(* Logix 5000 AddOnInstructionDefinition export Banner_IC70_PDIO_v4; software revision 33.03 *)

TYPE Banner_IC70_16P_PD_v4 :   // UDT that records the converted prcoess data.
STRUCT
   DTI : SINT[2];   // Data Transfer In
   DTO : SINT[2];   // Data Transfer Out
   PDI : Banner_IC70_16P_PDI_v4;   // Process Data In
   PDO : Banner_IC70_16P_PDO_v4;   // Process Data Out
END_STRUCT
END_TYPE

TYPE Banner_IC70_16P_PDI_v4 :
STRUCT
   C1_In : BOOL;   // Channel's current state: 0=Inactive, 1=Active
   C2_In : BOOL;   // Channel's current state: 0=Inactive, 1=Active
   C3_In : BOOL;   // Channel's current state: 0=Inactive, 1=Active
   C4_In : BOOL;   // Channel's current state: 0=Inactive, 1=Active
   C5_In : BOOL;   // Channel's current state: 0=Inactive, 1=Active
   C6_In : BOOL;   // Channel's current state: 0=Inactive, 1=Active
   C7_In : BOOL;   // Channel's current state: 0=Inactive, 1=Active
   C8_In : BOOL;   // Channel's current state: 0=Inactive, 1=Active
   C9_In : BOOL;   // Channel's current state: 0=Inactive, 1=Active
   C10_In : BOOL;   // Channel's current state: 0=Inactive, 1=Active
   C11_In : BOOL;   // Channel's current state: 0=Inactive, 1=Active
   C12_In : BOOL;   // Channel's current state: 0=Inactive, 1=Active
   C13_In : BOOL;   // Channel's current state: 0=Inactive, 1=Active
   C14_In : BOOL;   // Channel's current state: 0=Inactive, 1=Active
   C15_In : BOOL;   // Channel's current state: 0=Inactive, 1=Active
   C16_In : BOOL;   // Channel's current state: 0=Inactive, 1=Active
END_STRUCT
END_TYPE

TYPE Banner_IC70_16P_PDO_v4 :
STRUCT
   C1_Out : BOOL;   // Channel's current state: 0=Off, 1=On
   C2_Out : BOOL;   // Channel's current state: 0=Off, 1=On
   C3_Out : BOOL;   // Channel's current state: 0=Off, 1=On
   C4_Out : BOOL;   // Channel's current state: 0=Off, 1=On
   C5_Out : BOOL;   // Channel's current state: 0=Off, 1=On
   C6_Out : BOOL;   // Channel's current state: 0=Off, 1=On
   C7_Out : BOOL;   // Channel's current state: 0=Off, 1=On
   C8_Out : BOOL;   // Channel's current state: 0=Off, 1=On
   C9_Out : BOOL;   // Channel's current state: 0=Off, 1=On
   C10_Out : BOOL;   // Channel's current state: 0=Off, 1=On
   C11_Out : BOOL;   // Channel's current state: 0=Off, 1=On
   C12_Out : BOOL;   // Channel's current state: 0=Off, 1=On
   C13_Out : BOOL;   // Channel's current state: 0=Off, 1=On
   C14_Out : BOOL;   // Channel's current state: 0=Off, 1=On
   C15_Out : BOOL;   // Channel's current state: 0=Off, 1=On
   C16_Out : BOOL;   // Channel's current state: 0=Off, 1=On
END_STRUCT
END_TYPE

ADD_ON_INSTRUCTION Banner_IC70_PDIO_v4   (* revision 4.0, vendor Banner Engineering *)
// Takes the raw SINT information and converts that data into actual information.
VAR_IN_OUT
   PD : Banner_IC70_16P_PD_v4; {required}
END_VAR
VAR_INPUT
   Byte_Swap : BOOL; {required}   // Swap the LSB and the MSB with each other.
END_VAR
VAR
   Temp_Measurement : DINT; {access None}
   Byte_Out : SINT[2]; {access None}
   Byte_In : SINT[2]; {access None}
END_VAR

ROUTINE Logic   (* ladder *)
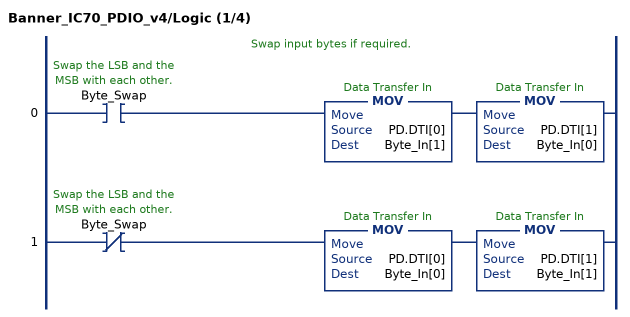
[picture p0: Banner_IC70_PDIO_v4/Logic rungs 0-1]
   // Swap input bytes if required.
   0: XIC(Byte_Swap)MOV(PD.DTI[0],Byte_In[1])MOV(PD.DTI[1],Byte_In[0]);
   1: XIO(Byte_Swap)MOV(PD.DTI[0],Byte_In[0])MOV(PD.DTI[1],Byte_In[1]);
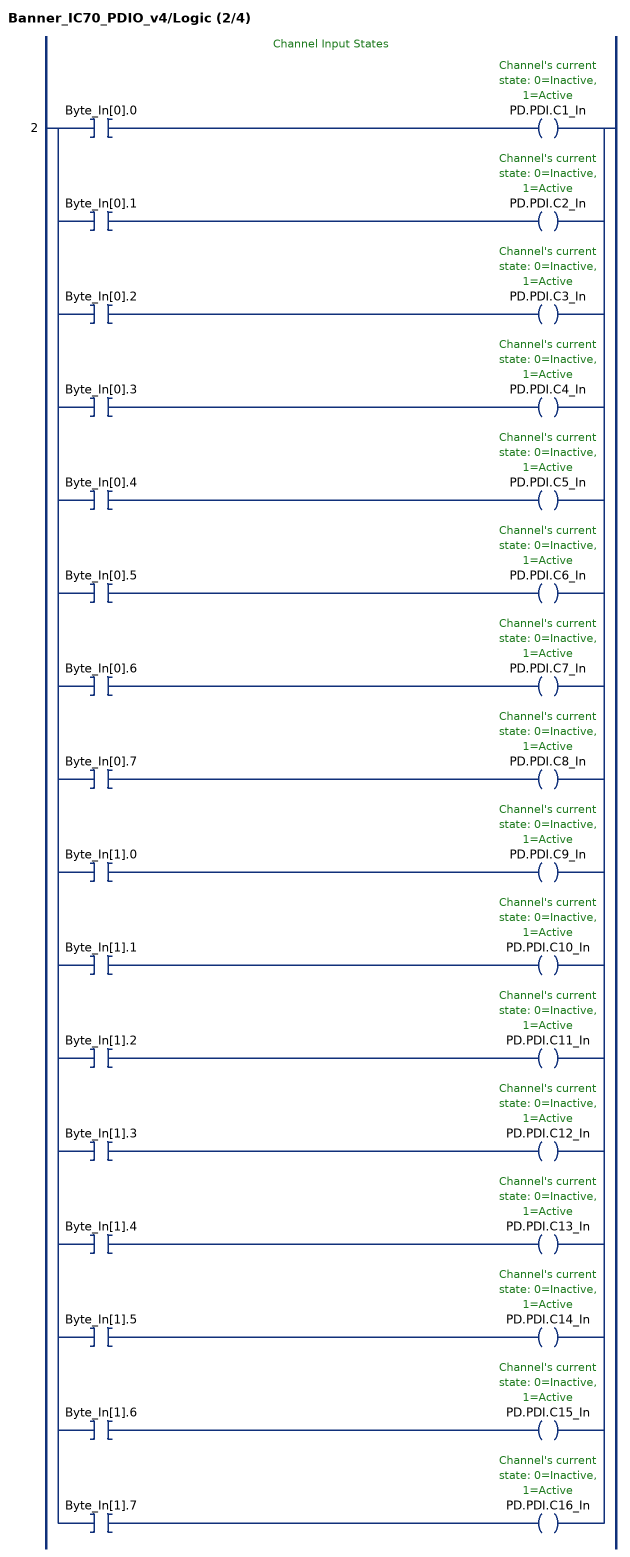
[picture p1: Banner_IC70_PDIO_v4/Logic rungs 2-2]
   // Channel Input States
   2: [XIC(Byte_In[0].0) OTE(PD.PDI.C1_In) ,XIC(Byte_In[0].1) OTE(PD.PDI.C2_In) ,XIC(Byte_In[0].2) OTE(PD.PDI.C3_In) ,XIC(Byte_In[0].3) OTE(PD.PDI.C4_In) ,XIC(Byte_In[0].4) OTE(PD.PDI.C5_In) ,XIC(Byte_In[0].5) OTE(PD.PDI.C6_In) ,XIC(Byte_In[0].6) OTE(PD.PDI.C7_In) ,XIC(Byte_In[0].7) OTE(PD.PDI.C8_In) ,XIC(Byte_In[1].0) OTE(PD.PDI.C9_In) ,XIC(Byte_In[1].1) OTE(PD.PDI.C10_In) ,XIC(Byte_In[1].2) OTE(PD.PDI.C11_In) ,XIC(Byte_In[1].3) OTE(PD.PDI.C12_In) ,XIC(Byte_In[1].4) OTE(PD.PDI.C13_In) ,XIC(Byte_In[1].5) OTE(PD.PDI.C14_In) ,XIC(Byte_In[1].6) OTE(PD.PDI.C15_In) ,XIC(Byte_In[1].7) OTE(PD.PDI.C16_In) ];
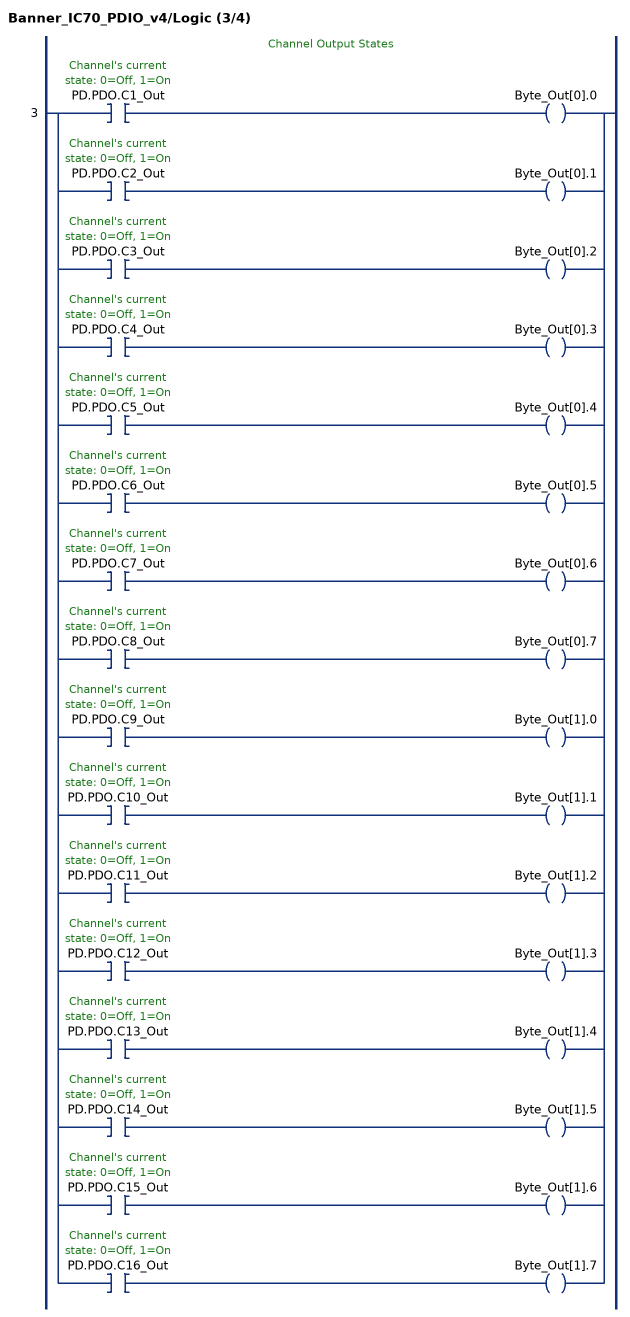
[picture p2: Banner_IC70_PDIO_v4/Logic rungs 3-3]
   // Channel Output States
   3: [XIC(PD.PDO.C1_Out) OTE(Byte_Out[0].0) ,XIC(PD.PDO.C2_Out) OTE(Byte_Out[0].1) ,XIC(PD.PDO.C3_Out) OTE(Byte_Out[0].2) ,XIC(PD.PDO.C4_Out) OTE(Byte_Out[0].3) ,XIC(PD.PDO.C5_Out) OTE(Byte_Out[0].4) ,XIC(PD.PDO.C6_Out) OTE(Byte_Out[0].5) ,XIC(PD.PDO.C7_Out) OTE(Byte_Out[0].6) ,XIC(PD.PDO.C8_Out) OTE(Byte_Out[0].7) ,XIC(PD.PDO.C9_Out) OTE(Byte_Out[1].0) ,XIC(PD.PDO.C10_Out) OTE(Byte_Out[1].1) ,XIC(PD.PDO.C11_Out) OTE(Byte_Out[1].2) ,XIC(PD.PDO.C12_Out) OTE(Byte_Out[1].3) ,XIC(PD.PDO.C13_Out) OTE(Byte_Out[1].4) ,XIC(PD.PDO.C14_Out) OTE(Byte_Out[1].5) ,XIC(PD.PDO.C15_Out) OTE(Byte_Out[1].6) ,XIC(PD.PDO.C16_Out) OTE(Byte_Out[1].7) ];
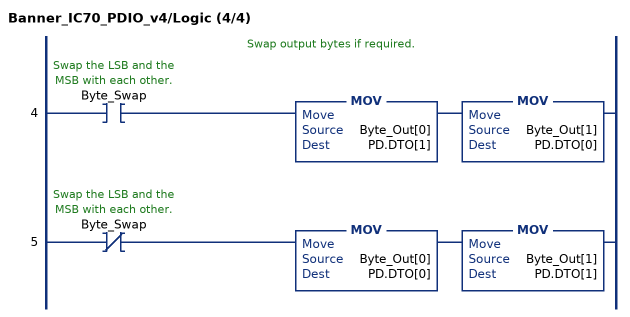
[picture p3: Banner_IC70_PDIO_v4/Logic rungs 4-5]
   // Swap output bytes if required.
   4: XIC(Byte_Swap)MOV(Byte_Out[0],PD.DTO[1])MOV(Byte_Out[1],PD.DTO[0]);
   5: XIO(Byte_Swap)MOV(Byte_Out[0],PD.DTO[0])MOV(Byte_Out[1],PD.DTO[1]);
END_ROUTINE
END_ADD_ON_INSTRUCTION
